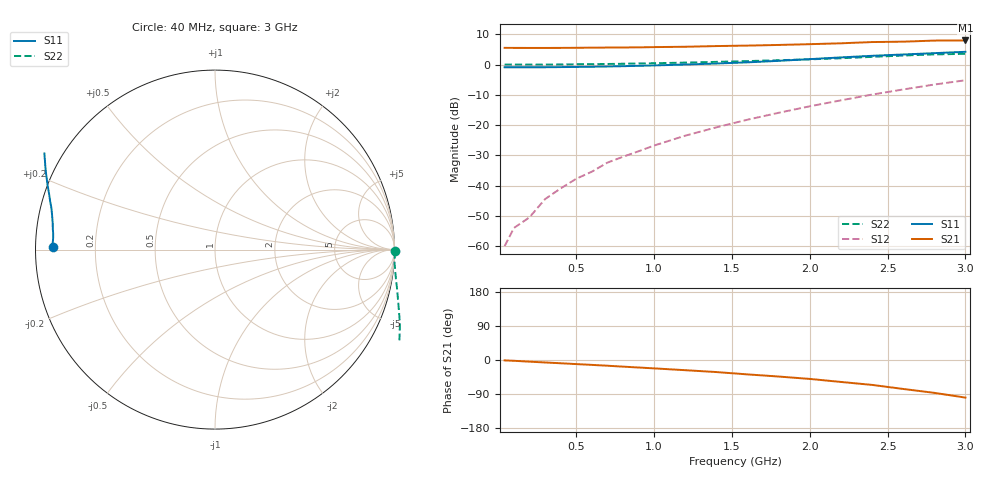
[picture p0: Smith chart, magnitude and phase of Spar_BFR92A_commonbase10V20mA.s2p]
! Filename:  BFR92ACJ.S2P  Version:  2.0
! NXP part #: BFR92A  Date: Jul 1990
! Bias condition: Vce=10V, Ic=20mA
! COMMON BASE
#  MHz  S  MA  R  50
! Freq  S11  S21  S12  S22
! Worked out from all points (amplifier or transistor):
!   21 points, 40 MHz to 3 GHz, reference 50 ohm
!   highest |S21| = 8.0 dB at 3 GHz (marker M1)
!   |S21| within 3 dB of that: start of sweep to end of sweep
!   unconditionally stable (mu >= 1): nowhere
!   at 300 MHz: K = -0.62, MSG = 25.0 dB, |S12| = -44.4 dB
!   at 1 GHz: K = -0.94, MSG = 16.3 dB, |S12| = -26.7 dB
!   at 3 GHz: K = -0.89, MSG = 6.6 dB, |S12| = -5.2 dB
40  0.905 179.1  1.893 -1.0  0.001 60.8  1.002 -0.6
100  0.905 178.0  1.892 -2.1  0.002 81.8  1.004 -1.3
200  0.904 176.1  1.889 -4.4  0.003 111.4  1.002 -2.9
300  0.906 174.3  1.888 -6.5  0.006 125.6  1.003 -4.4
400  0.911 172.7  1.892 -8.6  0.009 131.5  1.008 -5.8
500  0.916 170.8  1.898 -10.8  0.013 137.0  1.013 -7.3
600  0.923 169.1  1.909 -12.9  0.017 140.0  1.019 -8.7
700  0.932 167.2  1.916 -15.1  0.024 142.8  1.026 -10.2
800  0.943 165.4  1.923 -17.5  0.03 144.9  1.035 -11.7
900  0.956 163.8  1.931 -19.8  0.037 146.4  1.045 -13.4
1000  0.971 161.9  1.95 -22.1  0.046 147.4  1.055 -15.0
1200  1.004 158.5  1.975 -26.9  0.067 147.9  1.081 -18.5
1400  1.044 154.7  2.028 -31.8  0.092 146.8  1.112 -22.1
1600  1.091 150.6  2.065 -38.0  0.123 146.0  1.145 -26.2
1800  1.156 146.5  2.116 -43.6  0.16 143.6  1.184 -30.8
2000  1.233 142.2  2.18 -49.9  0.205 140.9  1.223 -36.2
2200  1.317 137.7  2.253 -57.9  0.257 137.5  1.276 -42.7
2400  1.4 132.8  2.363 -65.7  0.32 133.0  1.344 -49.9
2600  1.472 126.1  2.397 -76.4  0.389 128.2  1.415 -57.8
2800  1.549 117.8  2.499 -86.7  0.469 121.6  1.477 -66.0
3000  1.631 108.7  2.511 -99.2  0.552 114.9  1.51 -75.4
